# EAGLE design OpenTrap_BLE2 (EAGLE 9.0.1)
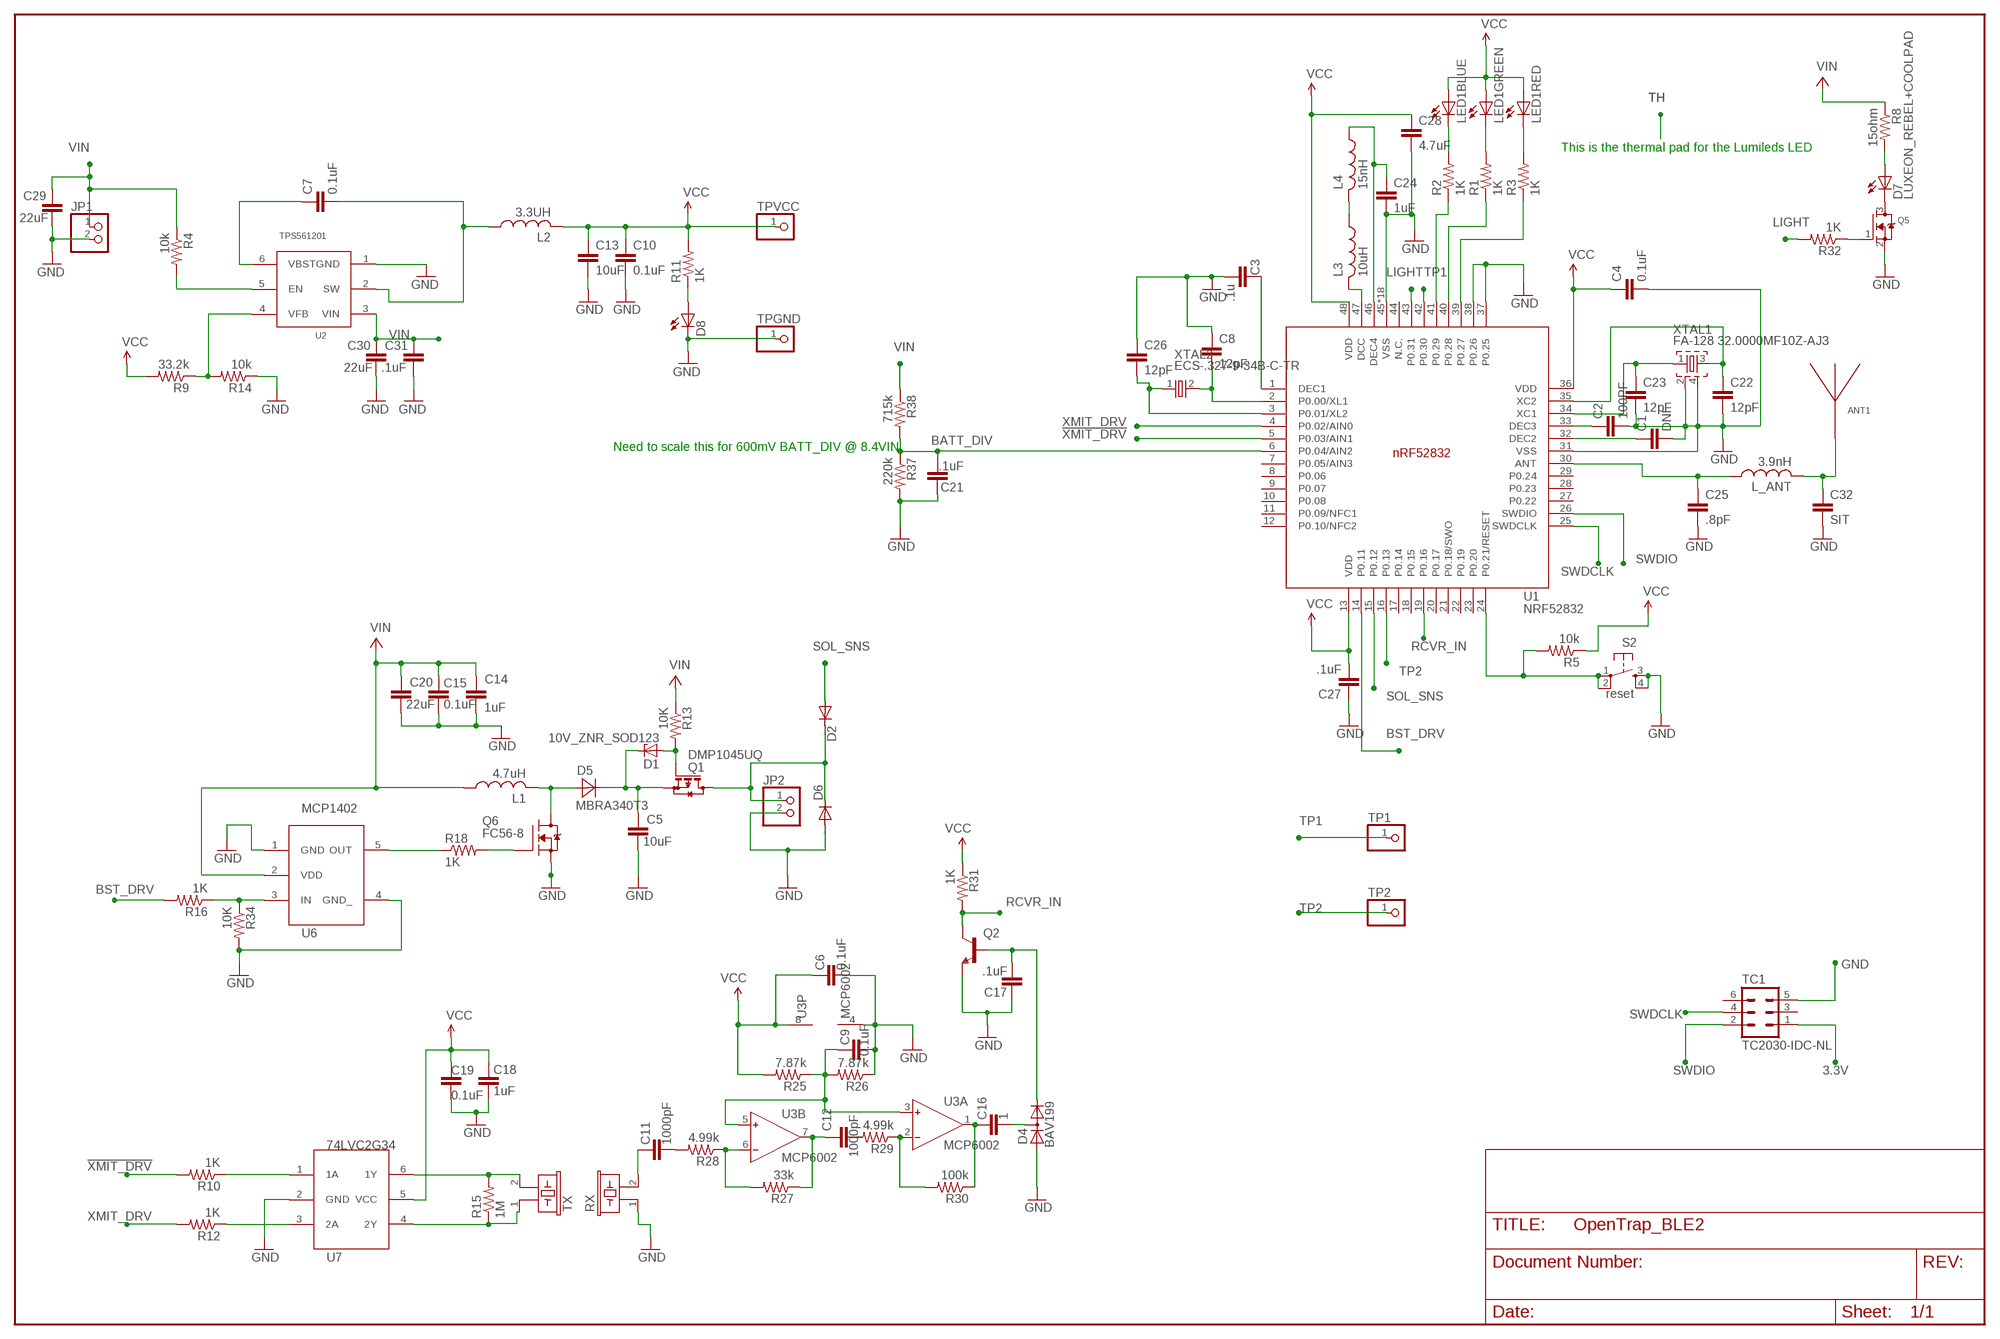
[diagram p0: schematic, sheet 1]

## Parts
ANT1  ANTENNA_QUARTER-WAVE_MONOPOLE_BEND_LEFT+1  [QWMP_BEND_LEFT_+1]
C1  DNI  C-EUC0402  [C0402]
C2  100PF  C-EUC0402  [C0402]
C3  .1u  C-EUC0402  [C0402]
C4  0.1uF  C-EUC0402  [C0402]
C5  10uF  CAP1210  [1210]
C6  0.1uF  CAP0805  [0805]
C7  0.1uF  CAP0805  [0805]
C8  12pF  C-EUC0402  [C0402]
C9  0.1uF  CAP0805  [0805]
C10  0.1uF  CAP0805  [0805]
C11  1000pF  CAP0805  [0805]
C12  1000pF  CAP0805  [0805]
C13  10uF  C-EUC0805  [C0805]
C14  1uF  CAP0805  [0805]
C15  0.1uF  CAP0805  [0805]
C16  1  CAP0805  [0805]
C17  .1uF  CAP0805  [0805]
C18  1uF  CAP0805  [0805]
C19  0.1uF  CAP0805  [0805]
C20  22uF  CAP1206  [1206]
C21  .1uF  CAP0805  [0805]
C22  12pF  C-EUC0402  [C0402]
C23  12pF  C-EUC0402  [C0402]
C24  1uF  C-EUC0603  [C0603]
C25  .8pF  C-EUC0402  [C0402]
C26  12pF  C-EUC0402  [C0402]
C27  .1uF  C-EUC0402  [C0402]
C28  4.7uF  C-EUC0603  [C0603]
C29  22uF  CAP1206  [1206]
C30  22uF  CAP1206  [1206]
C31  .1uF  CAP0805  [0805]
C32  SIT  C-EUC0402  [C0402]
D1  10V_ZNR_SOD123  [SOD123]
D2  DIODE-SOD123  [SOD123]
D4  BAV199  [SOT23]
D5  MBRA340T3  [SMA]
D6  DIODE-SOD123  [SOD123]
D7  LUXEON_REBEL+COOLPAD  [LUXEON_REBEL+COOLPAD]
D8  LEDCHIP-LED0805  [CHIP-LED0805]
JP1  PINHD-1X2  [1X02]
JP2  PINHD-1X2/90  [1X02/90]
L1  4.7uH  L-USV1  [ILHM2525]
L2  3.3UH  L-USSRN3015TA  [SRN3015TA]
L3  10uH  INDUCTOR_0402_M  [RESC0402_M]
L4  15nH  INDUCTOR_0201_M  [RESC0201_M]
L_ANT  3.9nH  INDUCTOR_0402_M  [RESC0402_M]
LED1  CLY6D-FKC  [CLY6D-FKC]
Q1  DMP1045UQ  BSS84  [SOT23]
Q2  MMBT2222ALT1-NPN-SOT23-BEC  [SOT23-BEC]
Q5  MOSFET-NREFLOW  [SOT23]
Q6  FC56-8  [FAIRCHILD56-8]
R1  1K  R-US_R0402  [R0402]
R2  1K  R-US_R0402  [R0402]
R3  1K  R-US_R0402  [R0402]
R4  10k  RESISTOR0805-RES  [0805]
R5  10k  RESISTOR0805-RES  [0805]
R8  15ohm  R-US_R1210  [R1210]
R9  33.2k  RESISTOR0805-RES  [0805]
R10  1K  RESISTOR0805-RES  [0805]
R11  1K  RESISTOR0805-RES  [0805]
R12  1K  RESISTOR0805-RES  [0805]
R13  10K  RESISTOR0805-RES  [0805]
R14  10k  RESISTOR0805-RES  [0805]
R15  1M  RESISTOR0805-RES  [0805]
R16  1K  RESISTOR0805-RES  [0805]
R18  1K  RESISTOR0805-RES  [0805]
R25  7.87k  RESISTOR0805-RES  [0805]
R26  7.87k  RESISTOR0805-RES  [0805]
R27  33k  RESISTOR0805-RES  [0805]
R28  4.99k  RESISTOR0805-RES  [0805]
R29  4.99k  RESISTOR0805-RES  [0805]
R30  100k  RESISTOR0805-RES  [0805]
R31  1K  RESISTOR0805-RES  [0805]
R32  1K  RESISTOR0805-RES  [0805]
R34  10K  RESISTOR0805-RES  [0805]
R37  220k  RESISTOR0805-RES  [0805]
R38  715k  RESISTOR0805-RES  [0805]
RX  EFBAA40D101  [EFBAA40D101]
S2  reset  TAC_SWITCHSMD  [TACTILE_SWITCH_SMD]
TC1  TC2030-IDC-NL  [TC2030-IDC-NL]
TP1  PINHD-1X1  [1X01]
TP2  PINHD-1X1  [1X01]
TPGND  PINHD-1X1  [1X01]
TPVCC  PINHD-1X1  [1X01]
TX  EFBAA40D101  [EFBAA40D101]
U1  NRF52832  [QFN40P600X600X90-48_N]
U2  TPS561201  [SOT23-6]
U3  MCP6002  AD8656RM  [MSOP08]
U6  MCP1402  [SOT23-DBV]
U7  74LVC2G34  [SOT23-6]
XTAL1  FA-128 32.0000MF10Z-AJ3  XTAL_32MHZ  [BT-XTAL_2016_N]
XTAL2  ECS-.327-9-34B-C-TR  XTAL_32KHZ  [XTAL_3215_N]

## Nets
3.3V [vcc]: C4.1 C6.2 C10.1 C13.1 C18.2 C19.2 C27.2 C28.1 L2.P$2 LED1.P$4(RED:A) LED1.P$5(GREEN:A) LED1.P$6(BLUE:A) R5.1 R9.2 R11.2 R25.2 R31.1 TC1.1 TPVCC.1 U1.13(VDD) U1.36(VDD) U1.48(VDD) U3.8(P:V+) U7.5(VCC) ; supply symbol labelled VCC
!XMIT_DRV: R10.2 U1.5(P0.03/AIN1)
BATT_DIV [GPIO]: C21.1 R37.1 R38.2 U1.6(P0.04/AIN2)
BST_DRV: R16.2 U1.14(P0.11)
GND [vcc]: C1.2 C2.2 C3.2 C4.2 C5.1 C6.1 C8.1 C9.1 C10.2 C13.2 C14.1 C15.1 C17.2 C18.1 C19.1 C20.1 C21.2 C22.2 C23.2 C24.2 C25.2 C26.1 C27.1 C28.2 C29.1 C30.1 C31.1 C32.2 D4.1(A) D6.A D8.C JP1.2 JP2.2 Q2.E Q5.2(S) Q6.1(S) Q6.2(S) Q6.3(S) R14.1 R26.1 R34.2 R37.2 RX.1 S2.3 S2.4 TC1.5 TPGND.1 U1.31(VSS) U1.37(P0.25) U1.38(P0.26) U1.45(VSS) U1.PAD(VSS) U1.PAD@VIA01(VSS) U1.PAD@VIA02(VSS) U1.PAD@VIA03(VSS) U1.PAD@VIA04(VSS) U1.PAD@VIA05(VSS) U1.PAD@VIA06(VSS) U1.PAD@VIA07(VSS) U1.PAD@VIA08(VSS) U1.PAD@VIA09(VSS) U1.PAD@VIA10(VSS) U1.PAD@VIA11(VSS) U1.PAD@VIA12(VSS) U1.PAD@VIA13(VSS) U1.PAD@VIA14(VSS) U1.PAD@VIA15(VSS) U1.PAD@VIA16(VSS) U2.1(GND) U3.4(P:V-) U6.1(GND) U6.4(GND_) U7.2(GND) XTAL1.2 XTAL1.4
LIGHT: R32.2 U1.43(P0.31)
N$1 [GPIO]: C22.1 U1.35(XC2) XTAL1.3
N$2 [GPIO]: C23.1 U1.34(XC1) XTAL1.1
N$3 [GPIO]: R18.1 U6.5(OUT)
N$4 [GPIO]: C1.1 U1.32(DEC2)
N$5 [GPIO]: C2.1 U1.33(DEC3)
N$6 [GPIO]: R16.1 R34.1 U6.3(IN)
N$7 [GPIO]: C8.2 U1.2(P0.00/XL1) XTAL2.2
N$8: Q6.4(G) R18.2
N$9 [GPIO]: C3.1 U1.1(DEC1)
N$10 [GPIO]: C26.2 U1.3(P0.01/XL2) XTAL2.1
N$11: R4.2 U2.5(EN)
N$12 [GPIO]: R15.1 TX.1 U7.4(2Y)
N$13 [GPIO]: R5.2 S2.1 S2.2 U1.24(P0.21/RESET)
N$14 [GPIO]: R15.2 TX.2 U7.6(1Y)
N$15: R3.1 U1.39(P0.27)
N$16: C11.2 RX.2
N$17 [GPIO]: C9.2 R25.1 R26.2 U3.3(A:IN+) U3.5(B:IN+)
N$18: C11.1 R28.2
N$19: R10.1 U7.1(1A)
N$20: D7.C D7.C@1(C) Q5.3(D)
N$21: C12.1 R29.2
N$22: Q5.1(G) R32.1
N$23: R1.1 U1.40(P0.28)
N$24 [boost]: D7.A D7.A@1(A) R8.2
N$25: R2.1 U1.41(P0.29)
N$26: LED1.P$3(RED:C) R3.2
N$27: R9.1 R14.2 U2.4(VFB)
N$28 [GPIO]: R27.2 R28.1 U3.6(B:IN-)
N$29: C7.1 U2.6(VBST)
N$30: LED1.P$2(GREEN:C) R1.2
N$31 [GPIO]: C12.2 R27.1 U3.7(B:OUT)
N$32: C7.2 L2.P$1 U2.2(SW)
N$33 [GPIO]: C16.2 R30.1 U3.1(A:OUT)
N$34 [GPIO]: R29.1 R30.2 U3.2(A:IN-)
N$35 [GPIO]: D2.C D6.C JP2.1 Q1.3(D)
N$36: C16.1 D4.3(AC)
N$37: LED1.P$1(BLUE:C) R2.2
N$38: D8.A R11.1
N$39: R12.1 U7.3(2A)
N$40 [vcc]: L3.1 L4.2
N$41 [GPIO]: C17.1 D4.2(C) Q2.B
N$42 [GPIO]: C5.2 D1.C D5.C Q1.2(S)
N$43 [vcc]: C24.1 L4.1 U1.46(DEC4)
N$44 [boost]: D5.A L1.2 Q6.5-8(D)
N$45 [GPIO]: D1.A Q1.1(G) R13.2
N$46 [vcc]: L3.2 U1.47(DCC)
N$49 [vcc]: C25.1 L_ANT.1 U1.30(ANT)
N$50 [vcc]: ANT1.P$1 C32.1 L_ANT.2
RCVR_IN: Q2.C R31.2 U1.19(P0.16)
SOL_SNS: D2.A U1.15(P0.12)
SWDCLK [GPIO]: TC1.4 U1.25(SWDCLK)
SWDIO [GPIO]: TC1.2 U1.26(SWDIO)
TP1: TP1.1 U1.42(P0.30)
TP2: TP2.1 U1.16(P0.13)
VIN [boost]: C14.2 C15.2 C20.2 C29.2 C30.2 C31.2 JP1.1 L1.1 R4.1 R8.1 R13.1 R38.1 U2.3(VIN) U6.2(VDD)
XMIT_DRV [GPIO]: R12.2 U1.4(P0.02/AIN0)
Unconnected: TC1.3 TC1.6 U1.7(P0.05/AIN3) U1.8(P0.06) U1.9(P0.07) U1.10(P0.08) U1.11(P0.09/NFC1) U1.12(P0.10/NFC2) U1.17(P0.14) U1.18(P0.15) U1.20(P0.17) U1.21(P0.18/SWO) U1.22(P0.19) U1.23(P0.20) U1.27(P0.22) U1.28(P0.23) U1.29(P0.24) U1.44(N.C.)

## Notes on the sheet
- This is the thermal pad for the Lumileds LED
- Need to scale this for 600mV BATT_DIV @ 8.4VIN

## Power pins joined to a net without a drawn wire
TH: D7.TH D7.TH@1(TH) D7.TH@2(TH) D7.TH@3(TH) D7.TH@4(TH) D7.TH@5(TH) D7.TH@6(TH) D7.TH@7(TH) D7.TH@8(TH) D7.TH@9(TH) D7.TH@10(TH) D7.TH@11(TH) D7.TH@12(TH) D7.TH@13(TH) D7.TH@14(TH) D7.TH@15(TH) D7.TH@16(TH) D7.TH@17(TH) D7.TH@18(TH) D7.TH@19(TH) D7.TH@20(TH) D7.TH@21(TH) D7.TH@22(TH) D7.TH@23(TH) D7.TH@24(TH) D7.TH@25(TH) D7.TH@26(TH) D7.TH@27(TH) D7.TH@28(TH) D7.TH@29(TH) D7.TH@30(TH) D7.TH@31(TH) D7.TH@32(TH) D7.TH@33(TH) D7.TH@34(TH) D7.TH@35(TH)

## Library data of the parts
ANT1 = Nordic_misc:ANTENNA_QUARTER-WAVE_MONOPOLE_BEND_LEFT
C1 C4 C13 C24 C27 C28 = rcl:C-EU: CAPACITOR, European symbol; SPICEPREFIX: C
C2 C8 C23 C25 C26 C32 = rcl:C-EU: CAPACITOR, European symbol; DIEL: C0G; SPICEPREFIX: C
C3 = rcl:C-EU: CAPACITOR, European symbol; DIEL: x7r; SPICEPREFIX: C
C5-C7 C9-C12 C14-C21 C29-C31 = SparkFun:CAP: Capacitor
C22 = rcl:C-EU: CAPACITOR, European symbol; DIEL: c0g; SPICEPREFIX: C
D1 = Roger_lib:10V_ZNR_SOD123
D2 D6 = diode:DIODE-: DIODE
D4 = diode:BAV199: DIODE low-leakage double diode
D5 = diode:MBRA340T3: Surface Mount Schottky Power Rectifier
D7 = led-lumiled:LUXEON_REBEL+COOLPAD: LUXEON REBEL LED with cooling pads Display Layer Refence in Board for more information Stop and Cream Mask defined by Luxeon Rebel Footprint _customer.dxf; OC_FARNELL: unknown; OC_NEWARK: unknown
D8 = led:LED: LED
JP1 JP2 = pinhead:PINHD-1X2: PIN HEADER
L1 = Rogerlib:L-US: INDUCTOR, American symbol
L2 = Roger_lib:L-US: INDUCTOR, American symbol
L3 L4 = Nordic_misc:INDUCTOR: Generic chip inductor
L_ANT = Nordic_nRF:INDUCTOR: Generic chip inductor
LED1 = Roger_lib:CLY6D-FKC
Q1 = transistor-small-signal:BSS84: P-CHANNEL MOS FET
Q2 = transistor-neu-to92:*-NPN-: NPN Transistror
Q5 = adafruit:MOSFET-N: N-Channel Mosfet 2N7002E - 60V 260mA SOT23 [Digikey: 2N7002ET1GOSTR-ND] - REEL BSH103 - 30V 850mA SOT23 [Digikey: 568-5013-1-ND]
Q6 = testlibFC56-8:FC56-8
R1-R3 = rcl:R-US_: RESISTOR, American symbol; SPICEPREFIX: R
R4 R5 R9-R16 R18 R25-R32 R34 R37 R38 = SparkFun:RESISTOR: Resistor
R8 = rcl:R-US_: RESISTOR, American symbol
RX TX = buzzer:EFB?: Piezoelectric Acoustic Transducer; OC_FARNELL: unknown; OC_NEWARK: unknown
S2 = SparkFun:TAC_SWITCH: Momentary Switch Button commonly used for reset or general input. Spark Fun Electronics SKU : COM-00097
TC1 = TagConnect:TC2030-IDC: Tag-Connect In Circuit Programming & Debug Cable 6 Pin http://www.tag-connect.com
TP1 TP2 TPGND TPVCC = pinhead:PINHD-1X1: PIN HEADER
U1 = Nordic_nRF:NRF52832: nRF52832 Features Single chip, highly flexible, 2.4 GHz multi-protocol SoC 32-bit ARM Cortex-M4F Processor 1.7v to 3.6v operation 512kB flash + 64kB RAM Supports concurrent Bluetooth Smart/ANT protocol operation On-chip NFC tag for Out-of-Band (OOB) pairing Up to +4dBm output power -96dBm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
U2 = Roger_lib:TPS561201
U3 = analog-devices:AD8656: Low Noise, Precision CMOS Amplifier Source: http://www.analog.com/static/imported-files/data_sheets/AD8655_8656.pdf; MPN: AD8656ARMZ; OC_FARNELL: 1117887; OC_NEWARK: 34P3252
U6 = Roger_lib:MCP1402
U7 = Roger_lib:74LVC2G34
XTAL1 = Nordic_nRF:XTAL_32MHZ
XTAL2 = Nordic_nRF:XTAL_32KHZ

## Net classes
1 vcc: width 0.203 mm
2 GPIO: width 0.152 mm
3 boost: width 0.381 mm

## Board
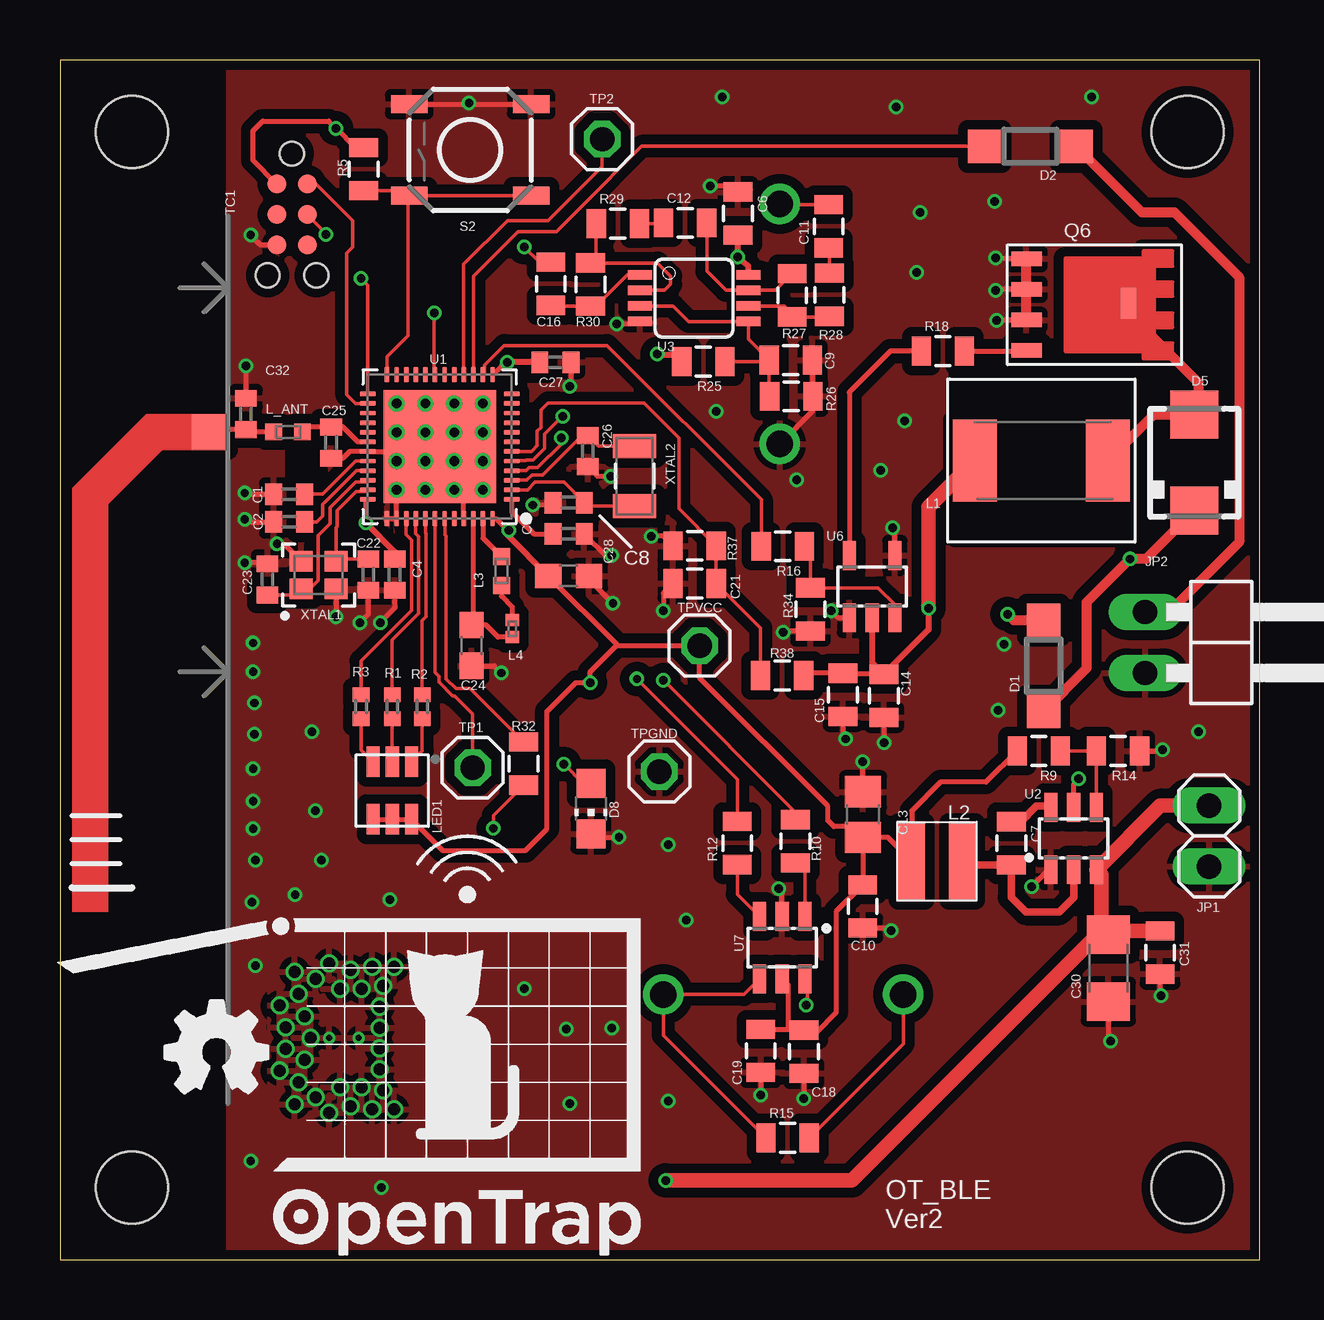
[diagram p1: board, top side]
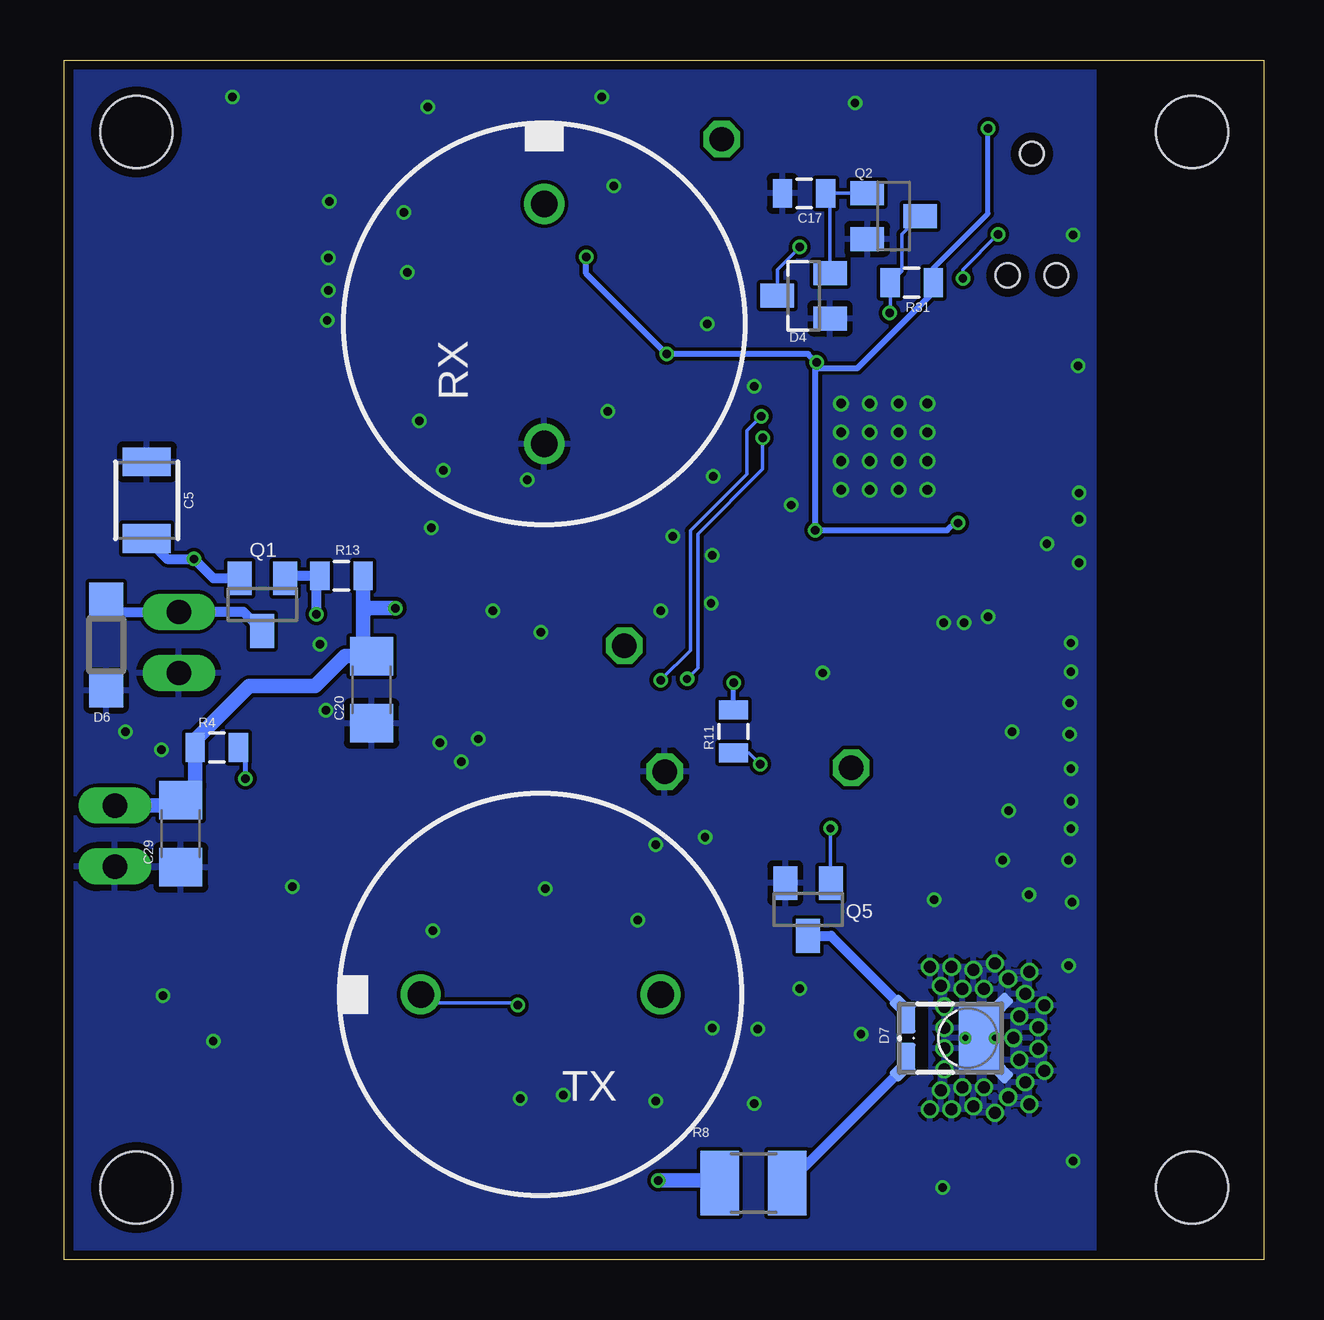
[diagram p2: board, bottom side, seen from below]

Size 50 x 50 mm. Coordinates in mm from the lower left corner, seen from the top.
Outline: 0,0 50,0 50,50 0,50 0,0
Copper layers (1*16): Top 0.035559375mm / dielectric 1.6mm / Bottom 0.035559375mm
Design rules "oshpark-2layer": minimum track width 6mil, minimum drill 10mil, track to track 6mil, track to pad 6mil, pad to pad 6mil, via to via 6mil, smd to smd 6mil, copper to edge 15mil, drill to drill 6mil, minimum pad ring 5mil, minimum via ring 5mil, stop-mask expansion 2.5mil, vias tented up to drill 0mil, thermal gap 10mil
Holes 3 mm at 3,47 3,3 47,3 47,47
tRestrict: area 9.8,32.5 to 10.4,33.8

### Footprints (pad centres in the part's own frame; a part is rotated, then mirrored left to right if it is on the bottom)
QWMP_BEND_LEFT_+1 = smd 1.5 x 1.5: P$1 0.75,0
C0402 = smd 0.7 x 0.9: 1 -0.65,0; 2 0.65,0
1210 = smd 1.2 x 2: 1 -1.6,0; 2 1.6,0
0805 = smd 0.8 x 1.2: 1 -0.9,0; 2 0.9,0
C0805 = smd 1.3 x 1.5: 1 -0.95,0; 2 0.95,0
1206 = smd 1.6 x 1.8: 1 -1.4,0; 2 1.4,0
C0603 = smd 1.1 x 1: 1 -0.85,0; 2 0.85,0
SOD123 = smd 1.4 x 1.4: A 1.9,0; C -1.9,0
SOT23 = smd 1 x 1.4: 1 -0.95,-1.1; 2 0.95,-1.1; 3 0,1.1
SMA = smd 2 x 2: A 2,0; C -2,0
LUXEON_REBEL+COOLPAD = smd 1.2 x 0.67: A 0.8,-2.51; C -0.8,-2.51 | smd 1 x 0.6 rotated 315: A@1 1.31,-2.75 | smd 1 x 0.6 rotated 225: C@1 -1.31,-2.75 | smd 2.8 x 1.77: TH 0,0.51 | smd 1 x 0.6 rotated 135: TH@1 -1.39,1.39 | smd 1 x 0.6 rotated 45: TH@2 1.39,1.39 | drill 0.5 pad 0.6: TH@3 2.971,-1.57; TH@4 2.971,-0.67; TH@5 2.85,0.23; TH@6 2.05,0.68; TH@7 2.05,-0.22; TH@8 2.171,-1.12; TH@9 2.764,2.575; TH@10 3.116,1.13; TH@11 2.461,1.687; TH@12 1.844,2.394; TH@13 0.9,2.15; TH@14 0,1.9; TH@15 0.45,2.95; TH@16 1.356,3.196; TH@17 1.31,-0.97; TH@18 0.43,-0.97; TH@21 -2.971,-1.57; TH@22 -2.971,-0.67; TH@23 -2.85,0.23; TH@24 -2.05,0.68; TH@25 -2.05,-0.22; TH@26 -2.171,-1.12; TH@27 -2.764,2.575; TH@28 -3.116,1.13; TH@29 -2.461,1.687; TH@30 -1.844,2.394; TH@31 -0.9,2.15; TH@32 -0.45,2.95; TH@33 -1.356,3.196; TH@34 -1.31,-0.97; TH@35 -0.43,-0.97 | drill 0.25 pad 0.4: TH@19 0,-0.095; TH@20 0,1.125
CHIP-LED0805 = smd 1.2 x 1.2: A 0,-1.05; C 0,1.05
1X02 = drill 1.016 long: 1 -1.27,0; 2 1.27,0
1X02/90 = drill 1.016 long: 1 -1.27,-3.81; 2 1.27,-3.81
ILHM2525 = smd 1.83 x 3.43: 1 -2.77,0; 2 2.77,0
SRN3015TA = smd 1.1 x 3.2: P$1 -1.05,0; P$2 1.05,0
RESC0402_M = smd 0.7 x 0.7: 1 -0.6,0; 2 0.6,0
RESC0201_M = smd 0.5 x 0.55: 1 -0.355,0; 2 0.355,0
CLY6D-FKC = smd 0.55 x 1.27: P$1 -0.8,-1.2; P$2 0,-1.2; P$3 0.8,-1.2; P$4 0.8,1.2; P$5 0,1.2; P$6 -0.8,1.2
SOT23-BEC = smd 1 x 1.4: B -0.95,-1.1; C 0,1.1; E 0.95,-1.1
FAIRCHILD56-8 = smd 0.61 x 1.27: 1 -1.91,-2.95; 2 -0.64,-2.95; 3 0.64,-2.95; 4 1.91,-2.95 | smd 1.27 x 0.635: 5-8 -0.05,1.3
R0402 = smd 0.6 x 0.7: 1 -0.5,0; 2 0.5,0
R1210 = smd 1.6 x 2.7: 1 -1.4,0; 2 1.4,0
EFBAA40D101 = drill 1.1 pad 1.676: 1 -5,0; 2 5,0
TACTILE_SWITCH_SMD = smd 1.524 x 0.762: 1 -2.54,1.905; 2 2.54,1.905; 3 -2.54,-1.905; 4 2.54,-1.905
TC2030-IDC-NL = smd 0.787 x 0.787: 1 -1.27,-0.635; 2 -1.27,0.635; 3 0,-0.635; 4 0,0.635; 5 1.27,-0.635; 6 1.27,0.635 | hole 0.991: -2.54,0; 2.54,1.016; 2.54,-1.016
1X01 = drill 1.016 octagon: 1 0,0
QFN40P600X600X90-48_N = smd 0.65 x 0.2: 1 -3,2.2; 2 -3,1.8; 3 -3,1.4; 4 -3,1; 5 -3,0.6; 6 -3,0.2; 7 -3,-0.2; 8 -3,-0.6; 9 -3,-1; 10 -3,-1.4; 11 -3,-1.8; 12 -3,-2.2; 25 3,-2.2; 26 3,-1.8; 27 3,-1.4; 28 3,-1; 29 3,-0.6; 30 3,-0.2; 31 3,0.2; 32 3,0.6; 33 3,1; 34 3,1.4; 35 3,1.8; 36 3,2.2 | smd 0.2 x 0.65: 13 -2.2,-3; 14 -1.8,-3; 15 -1.4,-3; 16 -1,-3; 17 -0.6,-3; 18 -0.2,-3; 19 0.2,-3; 20 0.6,-3; 21 1,-3; 22 1.4,-3; 23 1.8,-3; 24 2.2,-3; 37 2.2,3; 38 1.8,3; 39 1.4,3; 40 1,3; 41 0.6,3; 42 0.2,3; 43 -0.2,3; 44 -0.6,3; 45 -1,3; 46 -1.4,3; 47 -1.8,3; 48 -2.2,3 | smd 4.7 x 4.7: PAD 0,0 | drill 0.4: PAD@VIA01 -1.8,1.8; PAD@VIA02 -1.8,0.6; PAD@VIA03 -1.8,-0.6; PAD@VIA04 -1.8,-1.8; PAD@VIA05 -0.6,1.8; PAD@VIA06 -0.6,0.6; PAD@VIA07 -0.6,-0.6; PAD@VIA08 -0.6,-1.8; PAD@VIA09 0.6,1.8; PAD@VIA10 0.6,0.6; PAD@VIA11 0.6,-0.6; PAD@VIA12 0.6,-1.8; PAD@VIA13 1.8,1.8; PAD@VIA14 1.8,0.6; PAD@VIA15 1.8,-0.6; PAD@VIA16 1.8,-1.8
SOT23-6 = smd 0.55 x 1.2: 1 -0.95,-1.3; 2 0,-1.3; 3 0.95,-1.3; 4 0.95,1.3; 5 0,1.3; 6 -0.95,1.3
MSOP08 = smd 0.4 x 1: 1 -0.976,-2.263; 2 -0.326,-2.263; 3 0.324,-2.263; 4 0.974,-2.263; 5 0.974,2.262; 6 0.324,2.262; 7 -0.326,2.262; 8 -0.976,2.262
SOT23-DBV = smd 0.55 x 1.2: 1 -0.95,-1.3; 2 0,-1.3; 3 0.95,-1.3; 4 0.95,1.3; 5 -0.95,1.3
BT-XTAL_2016_N = smd 0.95 x 0.85: 1 -0.725,-0.575; 2 0.725,-0.575; 3 0.725,0.575; 4 -0.725,0.575
XTAL_3215_N = smd 1 x 1.8: 1 -1.25,0; 2 1.25,0

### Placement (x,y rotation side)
ANT1  7,34.5 180 top
C1  9.55,31.9 180 top
C2  9.55,30.75 180 top
C3  21.2,30.25 0 top
C4  13.95,28.55 270 top
C5  46.57,31.65 270 bottom
C6  28.26,43.6 270 top
C7  39.65,17.35 270 top
C8  21.2,31.55 0 top
C9  30.46,37.49 180 top
C10  33.46,14.72 270 top
C11  32.04,43.07 90 top
C12  26.06,43.21 0 top
C13  33.47,18.55 90 top
C14  34.34,23.5 90 top
C15  32.64,23.54 90 top
C16  20.46,40.67 270 top
C17  19.17,44.44 180 bottom
C18  31.01,8.66 90 top
C19  29.21,8.7 90 top
C20  37.2,23.75 90 bottom
C21  26.45,28.18 180 top
C22  12.85,28.55 270 top
C23  8.65,28.35 90 top
C24  17.15,25.6 270 top
C25  11.3,34.05 270 top
C26  22,33.7 90 top
C27  20.65,37.4 180 top
C28  21.2,28.5 0 top
C29  45.15,17.75 90 bottom
C30  43.7,12.15 90 top
C31  45.85,12.8 90 top
C32  7.75,35.25 90 top
D1  41,24.75 90 top
D2  40.45,46.4 180 top
D4  19.19,40.17 90 bottom
D5  47.28,33.21 90 top
D6  48.26,25.62 270 bottom
D7  12.35,9.23 270 bottom
D8  22.13,18.79 180 top
JP1  47.9,17.65 270 top
JP2  49.04,25.72 270 top
L1  40.91,33.3 0 top
L2  36.55,16.6 180 top
L3  18.4,28.7 90 top
L4  18.85,26.3 90 top
L_ANT  9.5,34.5 180 top
LED1  13.85,19.55 180 top
Q1  41.75,27.3 180 bottom
Q2  15.44,43.49 270 bottom
Q5  19,14.59 180 bottom
Q6  43.24,39.8 270 top
R1  13.85,23.05 270 top
R2  15.1,23.05 270 top
R3  12.55,23.05 270 top
R4  43.65,21.35 0 bottom
R5  12.65,45.45 270 top
R8  21.28,3.19 0 bottom
R9  40.8,21.2 180 top
R10  30.66,17.43 90 top
R11  22.11,22.01 90 bottom
R12  28.23,17.36 90 top
R13  38.45,28.5 180 bottom
R14  44.1,21.2 180 top
R15  30.33,5.07 0 top
R16  30.13,29.73 180 top
R18  36.8,37.87 0 top
R25  26.82,37.43 180 top
R26  30.48,35.98 180 top
R27  30.52,40.19 270 top
R28  32.07,40.21 90 top
R29  23.25,43.18 0 top
R30  22.12,40.64 90 top
R31  14.68,40.72 180 bottom
R32  19.32,20.67 90 top
R34  31.28,27.1 270 top
R37  26.45,29.75 180 top
R38  30.1,24.35 180 top
RX  30,39 90 bottom
S2  17.1,46.25 180 top
TC1  9.67,43.56 270 top
TP1  17.2,20.5 0 top
TP2  22.6,46.7 0 top
TPGND  24.98,20.34 0 top
TPVCC  26.66,25.59 0 top
TX  30.15,11.05 180 bottom
U1  15.83,33.88 180 top
U2  42.25,17.55 0 top
U3  26.43,40.07 270 top
U6  33.85,28.05 0 top
U7  30.1,13 180 top
U$1  [OTLOGO]  -0.35,-0.15 0 top
XTAL1  10.78,28.53 0 top
XTAL2  23.95,32.65 270 top

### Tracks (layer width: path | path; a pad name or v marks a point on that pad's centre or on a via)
3.3V  (via drill 0.35)
  Top 0.203: v12.75,30.7 12.75,31.6 U1.36 | U1.13 18.4,37.25 18.5,37.25 | U1.48 18.17,30.88 18.65,30.4 | 23.19,25.59 TPVCC.1 26.66,24.24 32,18.9 32,18.3 32.25,18.05 33.02,18.05 C13.1 | 23.19,25.59 22.1,24.5 v22.1,24.05 21.5,24.05 20.3,22.85 20.3,17.95 19.4,17.05 15.95,17.05 LED1.P$6 LED1.P$5 LED1.P$4 | C28.1 23.19,25.66 23.19,25.59 | R9.2 38.6,19.9 36.7,19.9 35.5,18.7 L2.P$2 34.5,17.6 C13.1 | C13.1 C10.1 32.35,14.51 32.35,10.3 31.55,9.5 31.49,9.56 C18.2 30.97,9.6 30.35,9.6 | C19.2 30.35,9.6 | U7.5 30.35,11.45 30.35,9.6 | R5.1 12.3,46.35 v11.5,47.15 11.2,47.45 8.45,47.45 8.05,47.05 8.05,45.81 TC1.1
  Top 0.254: C28.1 18.65,30.2 18.65,30.4 v18.7,30.4 | C27.2 v18.65,37.4 18.5,37.25 | C6.2 v28.25,41.8 28.69,41.41 U3.8 | R25.2 25.65,37.7 24.95,37.7 v24.9,37.75 | C4.1 13.95,29.5 v12.75,30.7
  Bottom 0.203: R11.2 v22.11,24.04 | v18.65,37.4 18.65,37.15 | R31.1 13.78,41.32 11.5,43.6 v11.5,47.15
  Bottom 0.254: v22.11,24.04 v22.1,24.05 | v12.75,30.7 12.8,30.7 12.85,30.75 13.2,30.4 v18.7,30.4 18.7,37.1 18.65,37.15 16.95,37.15 13.78,40.32 R31.1 | v18.65,37.4 19,37.75 v24.9,37.75 28.25,41.1 v28.25,41.8
!XMIT_DRV  (via drill 0.35)
  Top 0.152: U1.5 18.85,33.3 19.41,33.3 19.42,33.31 19.71,33.31 20.2,33.8 20.2,34.4 v20.95,35.15 | v25.15,24.15 30.66,18.64 R10.2
  Bottom 0.152: v20.95,35.15 21.55,34.55 21.55,32.73 23.91,30.38 23.91,25.39 v25.15,24.15
BATT_DIV
  Top 0.152: R38.2 29.2,26.32 C21.1 R37.1 25.8,31.3 25.8,34.25 24.35,35.7 20.75,35.7 20.65,35.7 20.35,35.7 20.05,35.4 20.05,34.68 19.89,34.53 19.89,33.93 19.65,33.68 U1.6
BST_DRV
  Top 0.152: U1.14 17.7,36.95 17.7,37.28 18.52,38.1 22.8,38.1 29.23,31.67 R16.2
GND  (via drill 0.35)
  Top 0.203: C25.2 11.8,33.4 12.08,33.68 U1.31 14.32,33.68 14.35,33.65 14.03,33.33 U1.PAD@VIA14 | U1.PAD@VIA13 U1.38 U1.37 | U1.45 16.83,31.68 U1.PAD@VIA05 | TC1.5 8.36,42.29 v7.95,42.7 | S2.4 16.9,48.16 | 16.9,48.16 S2.3 | v17.05,48.2 16.95,48.2 16.9,48.16 | C27.1 21.3,36.45 v21.25,36.4 | U3.4 24.07,39 v23.2,39 | C6.1 28.01,44.75 v27.1,44.75 | C9.1 31.36,36 R26.1 31.38,35.38 RX.1 | C8.1 20.45,31.45 v19.7,31.45 | C26.1 22.4,32.65 v22.95,32.65 | C3.2 22.75,29.35 v23,29.35 | C28.2 22.05,28.35 v23.05,27.35 | C21.2 25.15,27.77 v25.15,27.05 | R37.2 25.15,30.15 v24.65,30.15 | v7.7,31.95 7.75,31.9 C1.2 | v7.7,30.85 7.8,30.75 C2.2 | XTAL1.4 9.36,29.8 v9.05,29.84 | C23.2 8.6,29.05 v7.7,29.05 | XTAL1.2 v11.51,26.8 v11.5,26.8 | C22.2 12.85,26.9 v12.5,26.55 | C4.2 13.95,27.15 v13.35,26.55 | C24.2 18.1,24.75 v18.4,24.45 | R34.2 30.2,26.2 v30.15,26.15 | U6.1 32.45,26.75 v32.15,27.05 | C15.1 32.64,21.81 v32.75,21.7 | C14.1 34.34,21.79 v34.35,21.55 | C13.2 33.47,20.73 v33.45,20.75 | C19.1 29.21,6.99 v29.2,6.85 | C18.1 31.01,6.99 v31,6.7 | C10.2 34.53,13.82 v34.65,13.7 | U7.2 30.1,15.3 v29.95,15.45 | C32.2 v7.75,37.25 | R14.1 45.9,21.2 v45.95,21.25 | U2.1 41.2,16.25 v40.5,15.55 | C30.1 43.7,9.2 v43.8,9.1 | C31.1 45.85,11.05 v45.9,11 | U6.4 34.8,30.4 v34.7,30.5 | Q6.1 39.04,41.71 v39,41.75 | Q6.2 39.04,40.44 v39,40.4 | Q6.3 v39.06,39.16 v39.05,39.15 | U1.PAD U1.PAD@VIA11 | D8.C 22.27,17.6 v23.3,17.6
  Top 0.406: Q6.3 Q6.2 Q6.1
  other vias: 13.75,15 25.35,6.6 9.8,15.2 8.15,16.65 25.35,17.3 26.1,14.15 10.5,22 8.05,25.7 8.05,24.5 8.1,23.2 8.1,21.9 8.05,20.45 8.05,19.1 8.05,17.95 8,14.9 7.95,4.1 16.8,9.4 21.1,9.6 8.15,12.25 10.65,18.7 10.9,16.65 35.7,41.15 38.95,44.1 35.85,43.65 34.85,48.05 43,48.45 27.6,48.45 35.2,34.95 34.2,32.9 30.7,32.5 27.35,35.35 39.35,25.65 39.1,22.9 47.45,22 13.4,3 21.25,6.5 19.35,11.3 23,9.65
  pour Bottom: 7.1,51.35 7.1,-1.15 14.85,-0.75 53.35,-0.75 53.35,51.8
  pour Top (isolate 0.406): 7,53.1 7,-0.35 52.25,-0.35 52.25,53.1
LIGHT
  Top 0.152: R32.2 17.09,23.8 16.5,23.8 16.1,24.2 16.1,30.15 16.05,30.2 16.05,30.86 U1.43
N$1
  Top 0.152: C22.1 11.6,29.2 XTAL1.3 11.51,30.5 11.56,30.55 11.56,31.22 12.35,32.01 12.76,32.01 U1.35
N$2
  Top 0.152: C23.1 9.8,27.7 XTAL1.1 10.4,27.95 10.76,28.31 10.76,30.18 11.26,30.68 11.26,31.34 12.32,32.41 12.76,32.41 U1.34
N$3
  Top 0.203: R18.1 34.62,37.87 32.9,36.15 U6.5
N$4
  Top 0.152: U1.32 12.33,33.28 10.95,31.9 C1.1
N$5
  Top 0.152: U1.33 12.36,32.88 10.95,31.47 10.95,31 10.7,30.75 C2.1
N$6
  Top 0.152: R16.1 31.28,29.48 R34.1 34.1,28 34.8,27.3 U6.3
N$7
  Top 0.152: XTAL2.2 22,31.4 C8.2 21,32.4 19.8,32.4 19.48,32.08 U1.2
N$8
  Top 0.203: R18.2 40.27,37.87 Q6.4
N$9
  Top 0.203: U1.1 18.83,31.17 19.75,30.25 C3.1
N$10
  Top 0.152: U1.3 19.45,32.48 19.67,32.7 20.11,32.7 21.75,34.35 C26.2 22.45,33.9 XTAL2.1
N$11  (via drill 0.35)
  Top 0.203: U2.5 42.25,19.8 42.45,20 v42.45,20.05
  Bottom 0.203: v42.45,20.05 42.45,21.05 R4.2
N$12
  Top 0.152: U7.4 28.5,11.05 TX.1 25.15,9.35 R15.1
N$13
  Top 0.152: R5.2 14.36,44.55 14.5,44.4 | 14.5,44.4 S2.2 S2.1 | U1.24 13.63,37.63 14.5,38.5 14.5,44.4
N$14  (via drill 0.35)
  Top 0.152: U7.6 31.15,11.6 31.15,10.65 v31.1,10.6 | R15.2 35.15,8.99 TX.2
  Bottom 0.152: v31.1,10.6 31.2,10.7 34.8,10.7 TX.2
N$15
  Top 0.152: U1.39 14.43,30.22 14.65,30 14.65,27.05 12.55,24.95 R3.1
N$16
  Top 0.152: C11.2 30.03,43.97 RX.2
N$17
  Top 0.152: 29.56,37.4 C9.2 28.69,38.36 U3.5 26.2,39.1 25.55,39.75 U3.3 | 29.56,37.4 29.56,36 R26.2 | R25.1 29.53,37.43 29.56,37.4
N$18
  Top 0.152: C11.1 32.07,42.14 R28.2
N$19
  Top 0.152: U7.1 31.05,16.14 R10.1
N$20
  Bottom 0.406: Q5.3 18.05,13.49 D7.C@1
N$21
  Top 0.152: C12.1 25.13,43.18 R29.2
N$22  (via drill 0.35)
  Top 0.152: R32.1 18.07,18.52 v18.07,17.97
  Bottom 0.152: v18.07,17.97 18.07,15.71 Q5.1
N$23
  Top 0.152: R1.1 13.85,25.82 14.96,26.92 14.96,30.13 14.83,30.25 U1.40
N$24
  Bottom 0.406: D7.A@1 19.83,3.19 R8.2
N$25
  Top 0.152: R2.1 15.1,26.64 15.26,26.8 15.26,30.25 15.23,30.28 U1.41
N$26
  Top 0.152: LED1.P$3 12.55,21.25 R3.2
N$27
  Top 0.152: R9.1 R14.2 U2.4
N$28
  Top 0.152: R28.1 32.05,39.29 30.65,39.29 | 30.65,39.29 R27.2 | U3.6 30.19,39.75 30.65,39.29
N$29
  Top 0.305: C7.1 40.05,18.25 40.7,18.9 41.25,18.9 U2.6
N$30
  Top 0.152: LED1.P$2 R1.2
N$31
  Top 0.152: U3.7 | R27.1 29.83,40.4 28.8,40.4 U3.7 | C12.2 26.96,41.19 27.75,40.4 U3.7
N$32
  Top 0.305: U2.2 42.25,15.1 41.65,14.5 40.25,14.5 39.65,15.1 C7.2 37.75,16.45 L2.P$1
N$33
  Top 0.152: U3.1 23.65,41.05 22.34,39.74 R30.1 20.49,39.74 C16.2
N$34
  Top 0.152: R29.1 22.35,41.77 R30.2 24.91,41.54 25.45,41 25.45,40.65 25.2,40.4 U3.2
N$35
  Top 0.406: D2.C 45.1,43.65 46.45,43.65 49.15,40.95 49.15,29.9 46.24,26.99 JP2.1
  Bottom 0.406: Q1.3 42.54,26.99 JP2.1 47.73,26.99 D6.C
N$36  (via drill 0.35)
  Top 0.152: C16.1 19.98,41.57 v19.35,42.2
  Bottom 0.152: v19.35,42.2 20.29,41.26 D4.3
N$37
  Top 0.152: LED1.P$1 15.1,21.2 R2.2
N$38  (via drill 0.35)
  Top 0.152: D8.A 21.81,19.84 v21,20.65
  Bottom 0.152: R11.1 21.46,21.11 v21,20.65
N$39
  Top 0.152: R12.1 28.23,15.22 U7.3
N$40
  Top 0.203: L3.1 18.4,27.65 18.85,27.2 L4.2
N$41
  Bottom 0.152: D4.2 18.09,44.26 C17.1 Q2.B
N$42  (via drill 0.35)
  Top 0.406: D5.C 45.27,29.2 v44.6,29.2 42.8,27.4 42.8,24.65 D1.C
  Bottom 0.406: Q1.2 43.8,28.4 v44.6,29.2 45.72,29.2 C5.2
N$43
  Top 0.203: L4.1 18.26,25.94 17.75,26.45 C24.1 arc90 17.23,26.53 U1.46
N$44
  Top 0.406: Q6.5-8 44.54,39.46 47.45,36.55 47.45,35.38 D5.A 45.59,35.21 L1.2
N$45  (via drill 0.35)
  Top 0.406: v39.5,26.9 39.75,26.65 D1.A
  Bottom 0.406: Q1.1 40.7,28.5 R13.2 39.5,28.35 v39.5,26.9
N$46
  Top 0.203: U1.47 17.63,30.07 L3.2
N$49
  Top 0.203: U1.30 12.42,34.08 11.8,34.7 C25.1 10.3,34.7 L_ANT.1
N$50
  Top 0.203: L_ANT.2 7.85,34.5 C32.1 6.35,34.6 ANT1.P$1
RCVR_IN  (via drill 0.35)
  Top 0.152: v15.6,39.45 15.6,36.91 U1.19
  Bottom 0.152: Q2.C 15.1,42.73 15.1,41.2 R31.2 15.58,39.47 v15.6,39.45
SOL_SNS
  Top 0.152: D2.A 24.25,46.4 21.72,43.88 21.72,43.87 20.7,42.85 19.1,42.85 17.23,40.98 U1.15
SWDCLK  (via drill 0.35)
  Top 0.152: TC1.4 11.1,42.77 v11.1,42.75 v11.09,42.73 | v12.55,40.9 12.83,40.62 U1.25
  Bottom 0.152: v11.09,42.73 12.55,41.27 v12.55,40.9
SWDIO
  Top 0.152: U1.26 12.32,35.68 11.95,36.05 11.95,41.95 12.2,42.2 12.2,43.3 10.67,44.83 10.41,44.83 | 10.41,44.83 10.36,44.88 | TC1.2 10.41,44.83
TH
  pour Top: 8.9,13.2 14.15,13.2 14.65,12.7 14.65,5.7 14.25,5.3 9.95,5.3 8.7,5.3 8.7,13.25 8.9,13.25
  pour Bottom: 7.6,13.15 15.15,13.15 15.15,5.05 7.6,5.05
TP1
  Top 0.152: U1.42 15.63,24.47 15.79,24.3 15.79,24.07 16.37,23.5 16.45,23.5 17.2,22.75 TP1.1
TP2
  Top 0.152: TP2.1 22.6,45.55 20.35,43.3 18.65,43.3 16.83,41.48 U1.16
VIN  (via drill 0.35)
  Top 0.203: R38.1 31.09,24.44 C15.2 32.68,24.4 C14.2
  Top 0.254: v36.2,27.15 36.2,26.26 C14.2 33.85,24.89 U6.2
  Top 0.61: L1.1 36.2,31.36 v36.2,27.15 | v25.25,3.3 33,3.3 43.4,13.7 | 43.4,13.7 43.85,13.7 | 43.4,13.7 43.4,16.05 U2.3 45.87,18.92 JP1.1 | C30.2 43.85,13.7 | 43.85,13.7 C31.2
  Bottom 0.61: JP1.1 45.38,18.92 C29.2 44.55,19.75 R4.1 44.55,21.65 42.3,23.9 39.55,23.9 38.3,25.15 C20.2 37.55,25.5 37.55,26.95 | 37.55,26.95 R13.1 | v36.2,27.15 37.35,27.15 37.55,26.95 | R8.1 22.79,3.3 v25.25,3.3
XMIT_DRV  (via drill 0.35)
  Top 0.152: U1.4 19.42,32.88 19.55,33.01 19.91,33.01 20.9,34 v20.9,34.25 | v20.9,34.25 | v24.05,24.2 28.23,20.02 R12.2
  Bottom 0.152: v20.9,34.25 20.9,32.95 23.6,30.25 23.6,24.65 v24.05,24.2

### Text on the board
tNames: OT_BLE / Ver2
